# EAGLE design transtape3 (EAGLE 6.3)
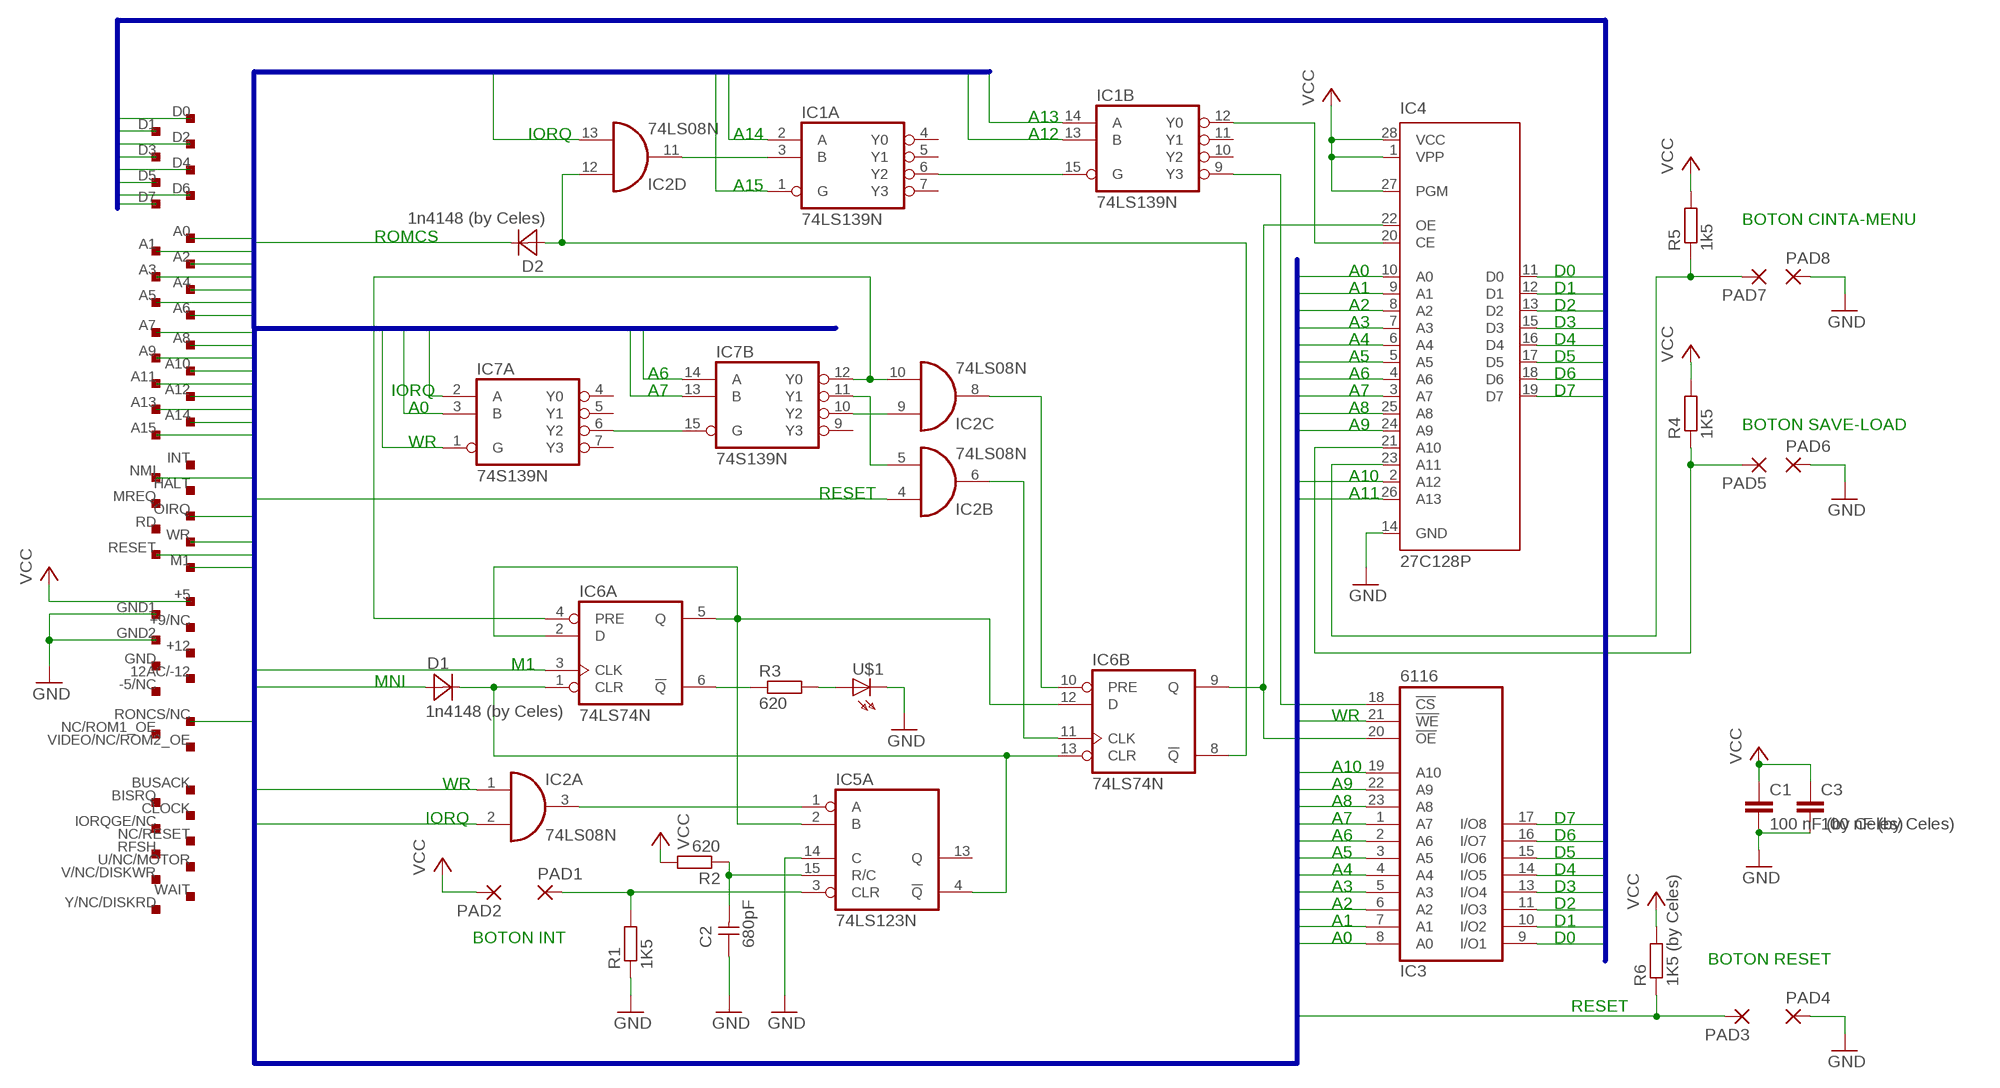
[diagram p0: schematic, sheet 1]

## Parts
C1  100 nF (by Celes)  C-EU050-025X075  [C050-025X075]
C2  680pF  CAPNP-5  [C-5]
C3  100 nF (by Celes)  C-EU050-025X075  [C050-025X075]
D1  1n4148 (by Celes)  DIODE-7,5  [D-7,5]
D2  1n4148 (by Celes)  DIODE-7,5  [D-7,5]
IC1  74LS139N  [DIL16]
IC2  74LS08N  [DIL14]
IC3  6116  6116P  [DIL24-6]
IC4  27C128P  [DIL28-6]
IC5  74LS123N  [DIL16]
IC6  74LS74N  [DIL14]
IC7  74S139N  [DIL16]
PAD1  1,6/0,9  [1,6/0,9]
PAD2  1,6/0,9  [1,6/0,9]
PAD3  1,6/0,9  [1,6/0,9]
PAD4  1,6/0,9  [1,6/0,9]
PAD5  1,6/0,9  [1,6/0,9]
PAD6  1,6/0,9  [1,6/0,9]
PAD7  1,6/0,9  [1,6/0,9]
PAD8  1,6/0,9  [1,6/0,9]
R1  1K5  R-EU_0207/10  [0207/10]
R2  620  R-EU_0207/10  [0207/10]
R3  620  R-EU_0207/10  [0207/10]
R4  1K5  R-EU_0207/10  [0207/10]
R5  1k5  R-EU_0207/10  [0207/10]
R6  1K5 (by Celes)  R-EU_0207/10  [0207/10]
U$1  LED3MM  [LED3MM]
U$2  SPECTRUM_V_1.0  [BUS_SPECTRUM_1.0]

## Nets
A0: IC3.8(A0) IC4.10(A0) IC7.3(A:B) U$2.A0
A1: IC3.7(A1) IC4.9(A1) U$2.A1
A2: IC3.6(A2) IC4.8(A2) U$2.A2
A3: IC3.5(A3) IC4.7(A3) U$2.A3
A4: IC3.4(A4) IC4.6(A4) U$2.A4
A5: IC3.3(A5) IC4.5(A5) U$2.A5
A6: IC3.2(A6) IC4.4(A6) IC7.14(B:A) U$2.A6
A7: IC3.1(A7) IC4.3(A7) IC7.13(B:B) U$2.A7
A8: IC3.23(A8) IC4.25(A8) U$2.A8
A9: IC3.22(A9) IC4.24(A9) U$2.A9
A10: IC3.19(A10) IC4.2(A12) U$2.A10
A11: IC4.26(A13) U$2.A11
A12: IC1.13(B:B) U$2.A12
A13: IC1.14(B:A) U$2.A13
A14: IC1.2(A:A) U$2.A14
A15: IC1.1(A:G) U$2.A15
D0: IC3.9(I/O1) IC4.11(D0) U$2.D0
D1: IC3.10(I/O2) IC4.12(D1) U$2.D1
D2: IC3.11(I/O3) IC4.13(D2) U$2.D2
D3: IC3.13(I/O4) IC4.15(D3) U$2.D3
D4: IC3.14(I/O5) IC4.16(D4) U$2.D4
D5: IC3.15(I/O6) IC4.17(D5) U$2.D5
D6: IC3.16(I/O7) IC4.18(D6) U$2.D6
D7: IC3.17(I/O8) IC4.19(D7) U$2.D7
GND: C1.2 C2.1 C3.2 IC4.14(GND) IC5.14(A:C) PAD4.1(P) PAD6.1(P) PAD8.1(P) R1.1 U$1.K(C) U$2.GND1 U$2.GND2
IORQ: IC2.2(A:I1) IC2.13(D:I1) IC7.2(A:A) U$2.OIRQ
M1: IC6.3(A:CLK) U$2.M1
MNI: D1.1(A) U$2.NMI
N$1: IC1.3(A:B) IC2.11(D:O)
N$2: IC1.6(A:Y2) IC1.15(B:G)
N$3: IC1.9(B:Y3) IC3.18(!CS)
N$4: IC1.12(B:Y0) IC4.20(CE)
N$5: C2.2 IC5.15(A:R/C) R2.1
N$7: IC7.6(A:Y2) IC7.15(B:G)
N$8: IC2.3(A:O) IC5.1(A:A)
N$10: IC5.2(A:B) IC6.2(A:D) IC6.5(A:Q) IC6.12(B:D)
N$11: IC5.3(A:CLR) PAD1.1(P) R1.2
N$12: IC2.5(B:I1) IC7.11(B:Y1)
N$13: IC2.9(C:I0) IC7.10(B:Y2)
N$15: D2.1(A) IC2.12(D:I0) IC6.8(B:!Q)
N$16: IC2.6(B:O) IC6.11(B:CLK)
N$17: D1.2(K) IC5.4(A:!Q) IC6.1(A:CLR) IC6.13(B:CLR)
N$18: IC2.8(C:O) IC6.10(B:PRE)
N$19: IC4.21(A10) PAD5.1(P) R4.1
N$21: IC2.10(C:I1) IC6.4(A:PRE) IC7.12(B:Y0)
N$22: IC6.6(A:!Q) R3.1
N$23: R3.2 U$1.A
N$25: IC3.20(!OE) IC4.22(OE) IC6.9(B:Q)
N$27: IC4.23(A11) PAD7.1(P) R5.1
RESET: IC2.4(B:I0) PAD3.1(P) R6.1 U$2.RESET
ROMCS: D2.2(K) U$2.RONCS/NC
VCC: C1.1 C3.1 IC4.1(VPP) IC4.27(PGM) IC4.28(VCC) PAD2.1(P) R2.2 R4.2 R5.2 R6.2 U$2.+5
WR: IC2.1(A:I0) IC3.21(!WE) IC7.1(A:G) U$2.WR
Unconnected: IC1.4(A:Y0) IC1.5(A:Y1) IC1.7(A:Y3) IC1.10(B:Y2) IC1.11(B:Y1) IC5.5(B:Q) IC5.6(B:C) IC5.7(B:R/C) IC5.9(B:A) IC5.10(B:B) IC5.11(B:CLR) IC5.12(B:!Q) IC5.13(A:Q) IC7.4(A:Y0) IC7.5(A:Y1) IC7.7(A:Y3) IC7.9(B:Y3) U$2.12AC/-12 U$2.+9/NC U$2.+12 U$2.-5/NC U$2.BISRQ U$2.BUSACK U$2.CLOCK U$2.GND U$2.HALT U$2.INT U$2.IORQGE/NC U$2.MREQ U$2.NC/RESET U$2.NC/ROM1_OE U$2.RD U$2.RFSH U$2.U/NC/MOTOR U$2.V/NC/DISKWR U$2.VIDEO/NC/ROM2_OE U$2.WAIT U$2.Y/NC/DISKRD

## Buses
WR,RESET,MNI,M1,IORQ,A[0..15],ROMCS
D[0..7]

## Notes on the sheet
- A13
- IORQ | A14 | A12
- A15
- BOTON CINTA-MENU
- ROMCS
- A0 | D0
- A1 | D1
- A2 | D2
- A3 | D3
- A4 | D4
- A5 | D5
- A6 | A6 | D6
- IORQ | A7 | A7 | D7
- A0 | A8
- A9 | BOTON SAVE-LOAD
- WR
- A10
- RESET | A11
- M1
- MNI
- WR
- A10
- WR | A9
- A8
- IORQ | A7 | D7
- A6 | D6
- A5 | D5
- A4 | D4
- A3 | D3
- A2 | D2
- A1 | D1
- BOTON INT | A0 | D0
- BOTON RESET
- RESET

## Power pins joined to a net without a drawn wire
GND: IC1.8(P:GND) IC2.7(P:GND) IC3.12(GND) IC5.8(P:GND) IC6.7(P:GND) IC7.8(P:GND)
VCC: IC1.16(P:VCC) IC2.14(P:VCC) IC3.24(VCC) IC5.16(P:VCC) IC6.14(P:VCC) IC7.16(P:VCC)

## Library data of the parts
C1 C3 = rcl:C-EU: CAPACITOR, European symbol
C2 = discrete:CAPNP-5
D1 D2 = discrete:DIODE-7,5
IC1 IC7 = 74xx-eu:74*139: Dual 2-line to 4-line DECODER/DEMULTIPLEXER
IC2 = 74xx-eu:74*08: Quad 2-input AND gate
IC3 = memory-idt:6116P: MEMORY
IC4 = microchip:27*128: CMOS EPROM 128 K (16 K x 8)
IC5 = 74xx-eu:74*123: Retriggerable monostable MULTIVIBRATOR
IC6 = 74xx-eu:74*74: Dual D type positive edge triggered FLIP FLOP, preset and clear
PAD1-PAD8 = wirepad:1,6/0,9: THROUGH-HOLE PAD
R1-R6 = rcl:R-EU_: RESISTOR, European symbol
U$1 = led:LED: LED
U$2 = spectrum:SPECTRUM_V_1.0

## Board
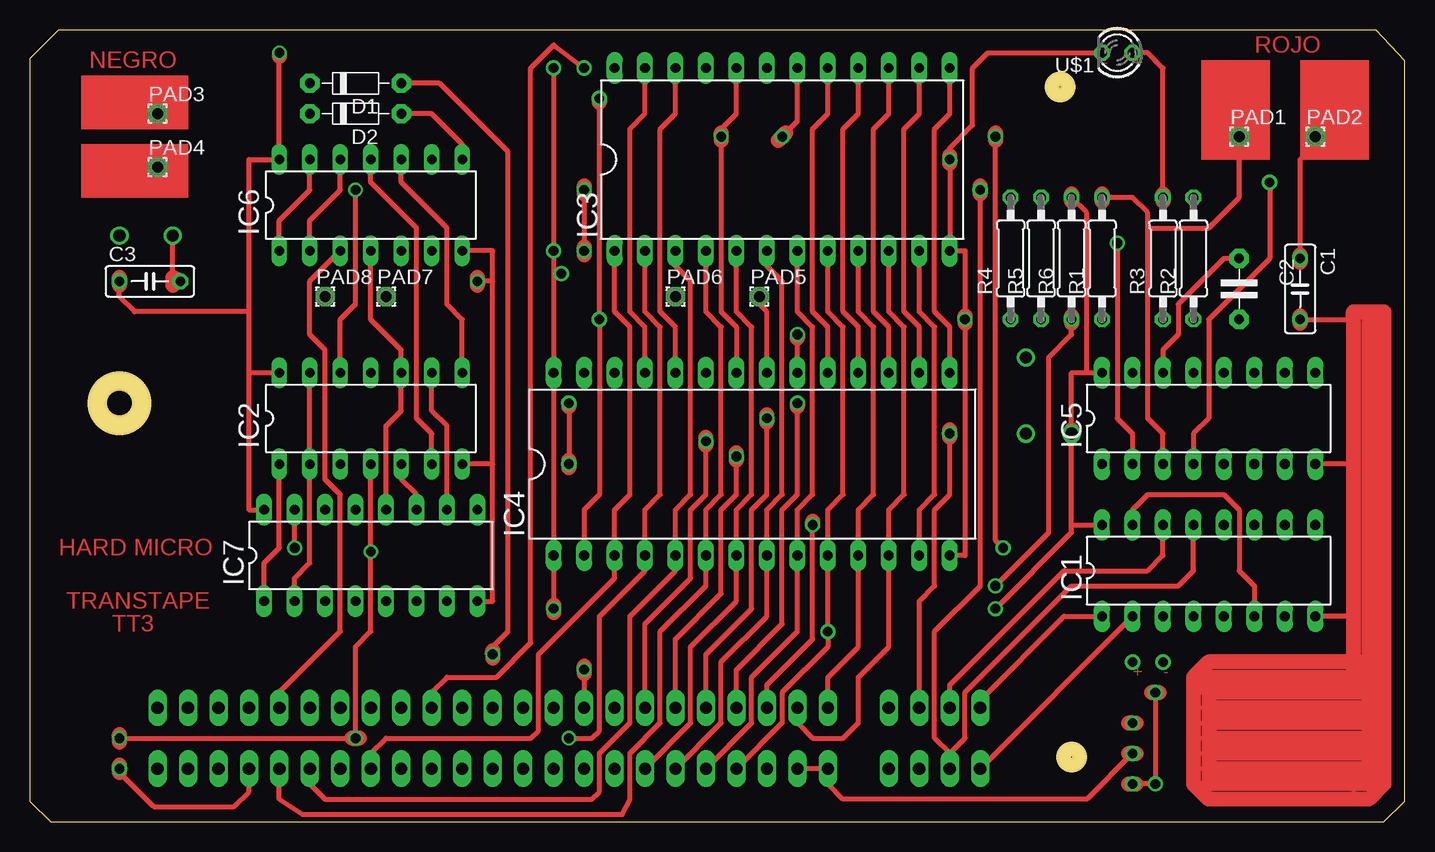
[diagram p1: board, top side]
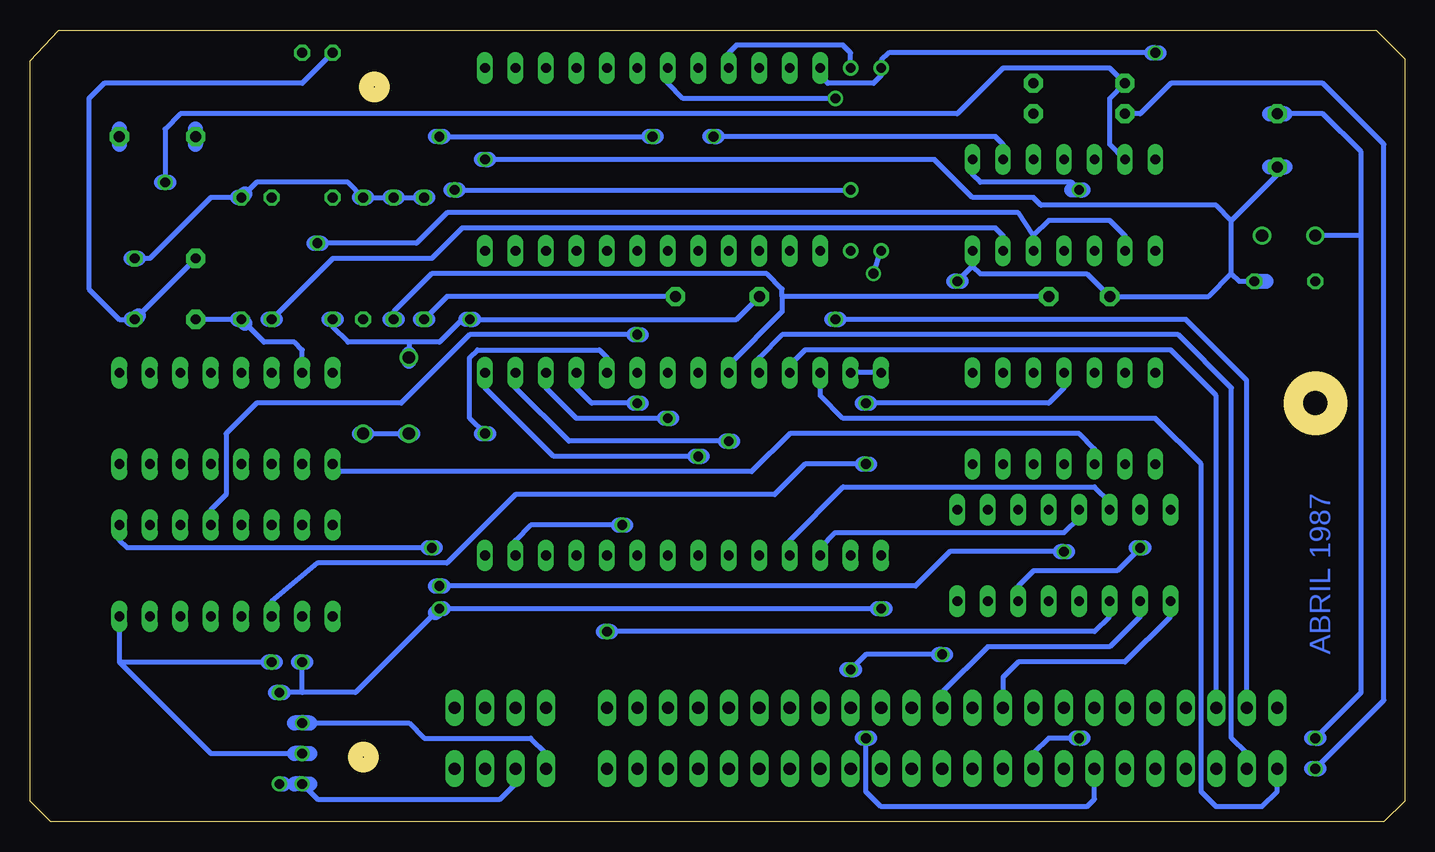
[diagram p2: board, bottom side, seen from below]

Size 114.61 x 66.04 mm. Coordinates in mm from the lower left corner, seen from the top.
Outline: 0,1.74 1.74,0 112.87,0 114.61,1.74 114.61,63.49 112.23,66.04 2.37,66.04 0,63.66 0,1.74
Outline: circle at 86.83,5.4 radius 0.64
Outline: circle at 85.88,61.28 radius 0.64
Outline: circle at 7.46,34.93 radius 1.62
Outline: circle at 7.46,34.93 radius 2.01
Copper layers (1*16): Top 0.035mm / dielectric 1.5mm / Bottom 0.035mm
Design rules "default": minimum track width 10mil, minimum drill 24mil, track to track 8mil, track to pad 8mil, pad to pad 8mil, via to via 8mil, smd to smd 8mil, copper to edge 40mil, drill to drill 8mil, minimum pad ring 10mil, minimum via ring 8mil, stop-mask expansion 4mil, vias tented up to drill 0mil, thermal gap 10mil

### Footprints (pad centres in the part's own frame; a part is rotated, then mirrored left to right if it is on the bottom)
C050-025X075 = drill 0.813 octagon: 1 -2.54,0; 2 2.54,0
C-5 = drill 0.813 pad 1.6 octagon: 1 -2.54,0; 2 2.54,0
D-7,5 = drill 0.813 pad 1.6 octagon: 1 -3.81,0; 2 3.81,0
DIL16 = drill 0.813 long: 1 -8.89,-3.81; 2 -6.35,-3.81; 3 -3.81,-3.81; 4 -1.27,-3.81; 5 1.27,-3.81; 6 3.81,-3.81; 7 6.35,-3.81; 8 8.89,-3.81; 9 8.89,3.81; 10 6.35,3.81; 11 3.81,3.81; 12 1.27,3.81; 13 -1.27,3.81; 14 -3.81,3.81; 15 -6.35,3.81; 16 -8.89,3.81
DIL14 = drill 0.8 long: 1 -7.62,-3.81; 2 -5.08,-3.81; 3 -2.54,-3.81; 4 0,-3.81; 5 2.54,-3.81; 6 5.08,-3.81; 7 7.62,-3.81; 8 7.62,3.81; 9 5.08,3.81; 10 2.54,3.81; 11 0,3.81; 12 -2.54,3.81; 13 -5.08,3.81; 14 -7.62,3.81
DIL24-6 = drill 0.813 long: 1 -13.97,-7.62; 2 -11.43,-7.62; 3 -8.89,-7.62; 4 -6.35,-7.62; 5 -3.81,-7.62; 6 -1.27,-7.62; 7 1.27,-7.62; 8 3.81,-7.62; 9 6.35,-7.62; 10 8.89,-7.62; 11 11.43,-7.62; 12 13.97,-7.62; 13 13.97,7.62; 14 11.43,7.62; 15 8.89,7.62; 16 6.35,7.62; 17 3.81,7.62; 18 1.27,7.62; 19 -1.27,7.62; 20 -3.81,7.62; 21 -6.35,7.62; 22 -8.89,7.62; 23 -11.43,7.62; 24 -13.97,7.62
DIL28-6 = drill 0.813 long: 1 -16.51,-7.62; 2 -13.97,-7.62; 3 -11.43,-7.62; 4 -8.89,-7.62; 5 -6.35,-7.62; 6 -3.81,-7.62; 7 -1.27,-7.62; 8 1.27,-7.62; 9 3.81,-7.62; 10 6.35,-7.62; 11 8.89,-7.62; 12 11.43,-7.62; 13 13.97,-7.62; 14 16.51,-7.62; 15 16.51,7.62; 16 13.97,7.62; 17 11.43,7.62; 18 8.89,7.62; 19 6.35,7.62; 20 3.81,7.62; 21 1.27,7.62; 22 -1.27,7.62; 23 -3.81,7.62; 24 -6.35,7.62; 25 -8.89,7.62; 26 -11.43,7.62; 27 -13.97,7.62; 28 -16.51,7.62
1,6/0,9 = drill 0.914 pad 1.6 octagon: 1 0,0
0207/10 = drill 0.813 octagon: 1 -5.08,0; 2 5.08,0
LED3MM = drill 0.813 octagon: A -1.27,0; K 1.27,0
BUS_SPECTRUM_1.0 = drill 1.016 long: 12AC/-12 12.7,2.54; +5 63.5,-2.54; +9/NC 60.96,-2.54; +12 15.24,2.54; -5/NC 20.32,2.54; A0 48.26,-2.54; A1 45.72,-2.54; A2 43.18,-2.54; A3 40.64,-2.54; A4 10.16,-2.54; A5 12.7,-2.54; A6 15.24,-2.54; A7 17.78,-2.54; A8 5.08,2.54; A9 2.54,-2.54; A10 2.54,2.54; A11 0,-2.54; A12 66.04,-2.54; A13 66.04,2.54; A14 68.58,-2.54; A15 68.58,2.54; BISRQ 22.86,-2.54; BUSACK 5.08,-2.54; CLOCK 50.8,-2.54; D0 55.88,2.54; D1 53.34,2.54; D2 50.8,2.54; D3 43.18,2.54; D4 40.64,2.54; D5 45.72,2.54; D6 48.26,2.54; D7 63.5,2.54; GND 35.56,-2.54; GND1 55.88,-2.54; GND2 53.34,-2.54; HALT 33.02,2.54; INT 38.1,2.54; IORQGE/NC 38.1,-2.54; M1 10.16,2.54; MREQ 30.48,2.54; NC/RESET 0,2.54; NC/ROM1_OE 60.96,2.54; NMI 35.56,2.54; OIRQ 27.94,2.54; RD 25.4,2.54; RESET 20.32,-2.54; RFSH 7.62,2.54; RONCS/NC 7.62,-2.54; U/NC/MOTOR 25.4,-2.54; V/NC/DISKWR 27.94,-2.54; VIDEO/NC/ROM2_OE 33.02,-2.54; WAIT 17.78,2.54; WR 22.86,2.54; Y/NC/DISKRD 30.48,-2.54

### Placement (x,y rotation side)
C1  105.88,44.45 270 top
C2  100.8,44.45 270 top
C3  9.99,45.09 0 top
D1  27.14,61.59 180 top
D2  27.14,59.05 180 top
IC1  98.26,20.95 0 top
IC2  28.41,33.66 0 top
IC3  62.7,55.25 0 top
IC4  60.16,29.84 0 top
IC5  98.26,33.66 0 top
IC6  28.41,51.44 0 top
IC7  28.41,22.22 0 top
PAD1  100.8,57.15 0 top
PAD2  107.15,57.15 0 top
PAD3  10.63,59.05 0 top
PAD4  10.63,54.61 0 top
PAD5  60.8,43.82 0 top
PAD6  53.81,43.82 0 top
PAD7  29.68,43.82 0 top
PAD8  24.6,43.82 0 top
R1  89.37,46.99 90 top
R2  96.99,46.99 90 top
R3  94.45,46.99 90 top
R4  81.75,46.99 90 top
R5  84.29,46.99 90 top
R6  86.83,46.99 90 top
U$1  90.64,64.13 180 top
U$2  10.63,6.99 0 top

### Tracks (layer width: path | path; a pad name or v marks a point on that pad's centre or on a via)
A0  (via drill 0.81 pad 1.27)
  Top 0.406: U$2.A0 62.7,8.26 62.7,10.79 66.51,14.61 v66.51,15.88 IC4.10 66.51,26.04 67.78,27.3 67.78,41.27 66.51,42.55 IC3.8
  Bottom 0.406: 66.19,15.88 25.87,15.88 24.6,17.14 IC7.3
  Bottom 1.27: v66.51,15.88 66.19,15.88 66.83,15.88
A1
  Top 0.406: IC3.7 63.97,42.55 65.24,41.27 65.24,27.3 63.97,26.04 IC4.9 63.97,15.88 60.16,12.06 60.16,8.26 U$2.A1
A2
  Top 0.406: IC3.6 61.43,46.36 62.7,45.09 62.7,27.3 61.43,26.04 IC4.8 61.43,17.14 57.62,13.34 57.62,8.26 U$2.A2
A3
  Top 0.406: IC3.5 58.89,42.55 60.16,41.27 60.16,27.3 58.89,26.04 IC4.7 58.89,18.41 55.08,14.61 55.08,8.26 U$2.A3
A4
  Top 0.406: IC3.4 56.35,42.55 57.62,41.27 57.62,27.3 56.35,26.04 IC4.6 56.35,19.68 52.54,15.88 52.54,8.26 50,5.71 50,1.91 49.37,0.64 22.7,0.64 20.79,1.91 U$2.A4
A5
  Top 0.406: U$2.A5 23.33,3.17 24.6,1.91 46.83,1.91 47.46,2.54 47.46,5.71 50,8.26 50,17.14 53.81,20.95 IC4.5 | IC4.5 53.81,22.86 | IC4.5 53.81,26.04 55.08,27.3 55.08,45.09 53.81,46.36 IC3.3
A6  (via drill 0.81)
  Top 0.406: IC3.2 51.27,42.55 52.54,41.27 52.54,27.3 51.27,26.04 IC4.4 51.27,20.95 47.46,17.14 47.46,7.62 46.83,6.99 v44.92,6.99
  Bottom 0.406: IC7.14 24.6,26.67 25.87,27.94 46.83,27.94 51.27,23.49 IC4.4 | U$2.A6 25.87,1.91 26.5,1.27 43.65,1.27 44.92,2.54 v44.92,6.99
  Bottom 1.27: 44.6,6.99 v44.92,6.99 45.24,6.99
A7
  Top 0.406: IC3.1 48.73,42.55 50,41.27 50,27.3 48.73,26.04 IC4.3 48.73,20.32 42.38,13.97 42.38,7.62 41.75,6.99 29.68,6.99 28.41,5.71 U$2.A7
  Bottom 0.406: IC7.13 27.14,25.4 28.41,24.13 47.46,24.13 48.73,22.86 IC4.3
A8
  Top 0.406: IC3.23 51.27,59.05 50,57.79 50,42.55 51.27,41.27 IC4.25
  Bottom 0.406: IC4.25 51.27,38.1 50,39.37 19.52,39.37 15.71,35.56 U$2.A8
A9
  Top 0.406: IC3.22 53.81,59.05 52.54,57.79 52.54,42.55 53.81,41.27 IC4.24
  Bottom 0.406: IC4.24 53.81,38.73 51.91,40.64 18.88,40.64 14.44,36.2 14.44,6.99 13.17,5.71 U$2.A9
A10  (via drill 0.81 pad 1.27)
  Top 0.406: IC4.2 46.19,26.04 47.46,27.3 v47.46,41.91 47.46,60.01
  Top 1.27: v47.46,60.33 47.46,60.01
  Bottom 0.406: U$2.A10 13.17,36.83 18.25,41.91 47.14,41.91 | IC3.19 61.43,61.59 60.16,60.33 v47.46,60.33
  Bottom 1.27: v47.46,41.91 47.14,41.91 47.78,41.91
A11
  Bottom 0.406: IC4.26 48.73,35.56 46.83,33.66 20.79,33.66 16.98,29.84 16.98,2.54 15.71,1.27 11.9,1.27 10.63,2.54 U$2.A11
A12  (via drill 0.81 pad 1.27)
  Top 0.406: U$2.A12 76.67,5.71 | 76.67,5.71 77.94,6.99 77.94,10.79 86.83,19.68 95.72,19.68 96.99,20.95 IC1.13 | 76.67,5.71 75.4,6.99 75.4,15.88 79.21,19.68 79.21,52.39 v79.21,52.71 | 46.19,52.39 46.19,47.94
  Top 1.27: 46.19,53.02 v46.19,52.71 46.19,52.39 | v46.19,47.62 46.19,47.94 46.19,47.31 | 79.21,53.02 v79.21,52.71 79.21,52.39
  Bottom 0.406: 78.89,52.71 v46.19,52.71
  Bottom 1.27: v79.21,52.71 78.89,52.71 79.53,52.71
A13
  Top 0.406: U$2.A13 76.67,11.43 86.2,20.95 93.18,20.95 94.45,22.22 IC1.14
A14
  Top 0.406: U$2.A14 IC1.2
A15
  Top 0.406: U$2.A15 79.21,10.16 86.2,17.14 IC1.1
D0
  Top 0.406: U$2.D0 66.51,12.06 69.05,14.61 IC4.11 69.05,26.04 70.32,27.3 70.32,41.27 69.05,42.55 IC3.9
D1
  Top 0.406: U$2.D1 63.97,8.26 65.24,6.99 67.78,6.99 69.05,8.26 69.05,12.06 71.59,14.61 IC4.12 71.59,26.04 72.86,27.3 72.86,41.27 71.59,42.55 IC3.10
D2  (via drill 0.81 pad 1.27)
  Top 0.406: U$2.D2 61.43,11.43 65.24,15.24 v65.24,24.76 | IC4.13 74.13,26.04 75.4,27.3 75.4,41.27 74.13,42.55 IC3.11
  Top 1.27: v65.24,24.76 65.24,25.08
  Bottom 0.406: v65.24,24.76 65.56,24.76 72.86,24.76 74.13,23.49 IC4.13
  Bottom 1.27: 64.92,24.76 v65.24,24.76 65.56,24.76
D3  (via drill 0.81 pad 1.27)
  Top 0.406: IC3.13 76.67,59.05 75.4,57.79 75.4,42.55 76.67,41.27 IC4.15 | U$2.D3 53.81,15.24 57.62,19.05 57.62,26.04 58.89,27.3 58.89,30.16 v58.89,30.48
  Top 1.27: 58.89,30.8 v58.89,30.48 58.89,30.16
  Bottom 0.406: IC4.15 76.67,36.2 70.95,30.48 59.21,30.48 v58.89,30.48
  Bottom 1.27: 58.57,30.48 v58.89,30.48 59.21,30.48
D4  (via drill 0.81 pad 1.27)
  Top 0.406: IC3.14 74.13,59.05 72.86,57.79 72.86,42.55 74.13,41.27 IC4.16 | U$2.D4 51.27,16.51 55.08,20.32 55.08,26.04 56.35,27.3 56.35,31.43 v56.35,31.75
  Top 1.27: 56.35,32.07 v56.35,31.75 56.35,31.43
  Bottom 0.406: IC4.16 74.13,36.2 69.69,31.75 56.67,31.75 v56.35,31.75
  Bottom 1.27: 56.03,31.75 v56.35,31.75 56.67,31.75
D5  (via drill 0.81 pad 1.27)
  Top 0.406: IC3.15 71.59,59.05 70.32,57.79 70.32,42.55 71.59,41.27 IC4.17 | U$2.D5 56.35,13.97 60.16,17.78 60.16,26.04 61.43,27.3 61.43,33.34 v61.43,33.66
  Top 1.27: 61.43,33.97 v61.43,33.66 61.43,33.34
  Bottom 0.406: IC4.17 71.59,36.2 69.05,33.66 61.75,33.66 v61.43,33.66
  Bottom 1.27: 61.11,33.66 v61.43,33.66 61.75,33.66
D6  (via drill 0.81 pad 1.27)
  Top 0.406: IC3.16 69.05,59.05 67.78,57.79 67.78,42.55 69.05,41.27 IC4.18 | U$2.D6 58.89,12.7 62.7,16.51 62.7,26.04 63.97,27.3 63.97,34.61
  Top 1.27: v63.97,34.93 63.97,34.61
  Bottom 0.406: IC4.18 69.05,36.2 67.78,34.93 64.29,34.93 v63.97,34.93
  Bottom 1.27: 63.65,34.93 v63.97,34.93 64.29,34.93
D7  (via drill 0.81 pad 1.27)
  Top 0.406: U$2.D7 74.13,18.41 75.4,19.68 75.4,26.04 76.67,27.3 76.67,32.07 v76.67,32.39 | IC3.17 66.51,59.05 65.24,57.79 65.24,42.55 66.51,41.27 IC4.19
  Top 1.27: 76.67,32.7 v76.67,32.39 76.67,32.07
  Bottom 0.406: v76.67,32.39 77.94,33.66 77.94,38.73 77.31,39.37 67.14,39.37 66.51,38.73 IC4.19
  Bottom 1.27: 76.35,32.39 v76.67,32.39 76.99,32.39
GND  (via drill 0.81, 0.81 pad 1.27, 1.02)
  Top 0.406: U$2.GND2 U$2.GND1 66.51,3.17 67.78,1.91 88.1,1.91 v91.91,5.71 | 110.33,17.14 IC1.8 | 110.33,29.84 IC5.8 | C1.2 110.33,41.91 | C2.1 99.53,46.99 95.72,43.18 95.72,40.64 94.45,39.37 IC5.14 | IC4.14 77.94,22.22 77.94,41.59 v77.94,41.91 | 77.94,42.23 77.94,47.62 IC3.12 76.67,54.93 | IC7.8 38.57,18.41 38.57,29.84 | 38.57,29.84 IC2.7 | 38.57,29.84 38.57,45.09 | 38.57,45.09 38.57,47.62 IC6.7 | 38.57,45.09 v37.3,45.09 | U$1.K 79.84,64.13 78.58,62.87 78.58,58.1 76.67,56.2 v76.67,55.25 | 11.9,45.4 v11.9,48.9
  Top 1.27: 98.26,4.45 98.26,3.17 110.33,3.17 | 98.26,6.99 98.26,5.71 | 98.26,9.53 98.26,8.26 | 98.26,10.79 98.26,12.06 110.33,12.06 | 111.59,12.06 110.33,12.06 | 111.59,12.06 111.59,10.79 | 111.59,10.79 111.59,9.53 | 111.59,8.26 111.59,6.99 | 111.59,5.71 111.59,4.45 | 111.59,4.45 111.59,3.17 110.33,3.17 | 111.59,4.45 110.33,3.17 | 111.59,4.45 98.26,4.45 | 98.26,5.71 98.26,4.45 | 111.59,5.71 98.26,5.71 | 111.59,6.99 111.59,5.71 | 111.59,6.99 98.26,6.99 | 98.26,8.26 98.26,6.99 | 111.59,8.26 98.26,8.26 | 111.59,9.53 111.59,8.26 | 111.59,9.53 98.26,9.53 | 98.26,10.79 98.26,9.53 | 111.59,10.79 98.26,10.79 | 110.33,12.06 111.59,10.79 | 110.33,13.34 98.26,13.34 96.99,12.06 96.99,3.17 98.26,1.91 111.59,1.91 112.87,3.17 112.87,13.34 | 110.33,13.34 110.33,17.14 110.33,29.84 110.33,41.91 110.33,42.55 111.59,42.55 | 111.59,42.55 112.87,42.55 112.87,13.34 | 110.33,13.34 110.33,12.06 | 110.33,13.34 112.87,13.34 | 111.59,12.06 112.87,13.34 | 111.59,42.55 111.59,12.06 | 91.59,5.71 v91.91,5.71 92.23,5.71 | v77.94,41.91 77.94,42.23 77.94,41.59 | 76.67,55.56 v76.67,55.25 76.67,54.93 | 37.3,45.4 v37.3,45.09 37.3,44.77 | C3.2 11.9,45.4 11.9,44.77 | 105.88,42.23 C1.2 105.88,41.59
  Bottom 0.406: 92.55,5.71 99.53,5.71 107.15,13.34 | 107.15,13.34 94.45,13.34 | IC1.8 107.15,13.34 | 106.2,41.91 107.15,41.91 109.69,44.45 109.69,60.33 108.42,61.59 91.91,61.59 U$1.K | 105.56,42.23 C2.1 | v37.3,45.09 36.03,46.36 | 36.03,46.36 IC6.7 | 36.03,46.36 35.4,45.72 26.5,45.72 PAD8.1 16.34,43.82 14.44,45.72 | 12.22,45.09 13.8,45.09 14.44,45.72 | 14.44,45.72 14.44,50.16 | 76.35,55.25 39.21,55.25 36.03,52.07 30.95,52.07 30.31,51.44 15.71,51.44 14.44,50.16 | PAD4.1 10.63,53.98 14.44,50.16 | PAD6.1 55.72,41.91 77.62,41.91 | 83.02,40.01 80.48,40.01 78.58,41.91 78.26,41.91 v77.94,41.91 | 83.02,40.01 88.1,40.01 89.37,41.27 R1.1 | 83.02,40.01 83.02,39.05
  Bottom 1.27: 91.28,5.71 v91.91,5.71 92.55,5.71 | 83.02,39.05 v83.02,38.73 83.02,38.42 | v76.67,55.25 76.35,55.25 76.99,55.25 | v77.94,41.91 77.62,41.91 78.26,41.91 | 36.98,45.09 v37.3,45.09 37.62,45.09 | 11.58,45.09 C3.2 12.22,45.09 | 105.56,42.23 C1.2 106.2,41.91 | 89.05,41.91 R1.1 89.69,41.91 | 9.99,54.61 PAD4.1 11.27,54.61
IORQ
  Top 0.406: IC7.2 22.06,20.32 23.33,21.59 IC2.2 IC2.13
  Bottom 0.406: IC7.2 22.06,17.14 24.6,14.61 34.76,14.61 38.57,10.79 U$2.OIRQ
M1
  Top 0.406: U$2.M1 20.79,10.79 25.87,15.88 25.87,27.3 24.6,28.57 24.6,39.37 23.33,40.64 23.33,45.09 IC6.3
MNI  (via drill 0.81)
  Top 0.406: D1.1 34.12,61.59 39.84,55.88 39.84,15.88 38.57,14.61 38.57,14.29 | 46.19,12.38 U$2.NMI
  Top 1.27: 46.19,13.02 v46.19,12.7 46.19,12.38 | v38.57,13.97 38.57,14.29 38.57,13.65
  Bottom 0.406: v38.57,13.97 38.89,13.97 44.92,13.97 v46.19,12.7
  Bottom 1.27: 45.87,12.7 v46.19,12.7 46.51,12.7 | 38.25,13.97 v38.57,13.97 38.89,13.97
N$1  (via drill 0.81 pad 1.27)
  Top 0.406: 44.92,34.61 44.92,30.16
  Top 1.27: v44.92,29.84 44.92,30.16 44.92,29.53 | v44.92,34.93 44.92,34.61
  Bottom 0.406: IC1.3 94.45,18.41 90.64,21.59 79.84,21.59 74.13,27.3 52.54,27.3 50,29.84 45.24,29.84 | 44.6,34.93 29.68,34.93 28.41,36.2 IC2.11
  Bottom 1.27: 44.6,29.84 v44.92,29.84 45.24,29.84 | v44.92,34.93 44.6,34.93 45.24,34.93
N$2
  Top 0.406: IC1.15 91.91,26.04 93.18,27.3 99.53,27.3 100.8,26.04 100.8,20.95 102.07,19.68 IC1.6
N$3  (via drill 0.81 pad 1.27)
  Top 0.406: v81.12,22.86 80.48,23.49 80.48,56.83 | 63.02,57.47 63.97,58.42 IC3.18
  Top 1.27: 80.48,57.47 v80.48,57.15 80.48,56.83 | v62.7,57.15 63.02,57.47 62.38,56.83
  Bottom 0.406: IC1.9 107.15,23.49 106.52,22.86 81.43,22.86 | 80.16,57.15 63.02,57.15 v62.7,57.15
  Bottom 1.27: 80.8,22.86 v81.12,22.86 81.43,22.86 | v80.48,57.15 80.16,57.15 80.8,57.15 | 62.38,57.15 v62.7,57.15 63.02,57.15
N$4  (via drill 0.81 pad 1.27)
  Top 0.406: IC4.20 63.97,40.32
  Top 1.27: v63.97,40.64 63.97,40.32
  Bottom 0.406: IC1.12 99.53,26.04 98.26,27.3 98.26,32.39 95.72,34.93 83.66,34.93 77.94,40.64 64.29,40.64 v63.97,40.64
  Bottom 1.27: 63.65,40.64 v63.97,40.64 64.29,40.64
N$5
  Bottom 0.406: 97.31,41.91 C2.2 | 96.67,41.59 95.09,40.01 92.55,40.01 91.91,39.37 IC5.15
  Bottom 1.27: 97.31,41.91 R2.1 96.67,41.59
N$6  (via drill 0.81)
  Top 1.27: 91.59,8.26 v91.91,8.26 92.23,8.26
  Bottom 0.406: 91.28,8.26 83.02,8.26 81.75,6.99 72.86,6.99 71.59,5.71
  Bottom 1.27: v91.91,8.26 91.28,8.26 92.55,8.26
N$7  (via drill 0.81 pad 1.27)
  Top 0.406: v22.06,22.86 IC7.15
  Bottom 0.406: IC7.6 32.22,19.68 30.95,20.95 23.96,20.95 v22.06,22.86
  Bottom 1.27: 21.74,22.86 v22.06,22.86 22.38,22.86
N$8
  Bottom 0.406: IC5.1 88.73,29.21 54.45,29.21 51.27,32.39 27.14,32.39 25.87,31.11 IC2.3
N$10  (via drill 0.81 pad 1.27)
  Top 0.406: IC5.2 91.91,32.39 90.64,33.66 v90.64,48.26 | IC6.2 23.33,50.16 25.87,52.71 IC6.12
  Bottom 0.406: 90.32,48.26 82.39,48.26 79.84,50.8 32.22,50.8 30.95,48.9 | 30.95,48.9 IC6.5 | 30.95,48.9 29.68,50.16 24.6,50.16 23.33,48.9 IC6.2
  Bottom 1.27: v90.64,48.26 90.32,48.26 90.96,48.26
N$11
  Top 0.406: PAD1.1 100.8,52.07 98.26,49.53 93.18,49.53 | R1.2 91.91,52.07 93.18,50.8 93.18,49.53 | 93.18,49.53 93.18,33.66 94.45,32.39 IC5.3
  Top 1.27: 89.37,52.39 R1.2 89.37,51.75
  Bottom 1.27: 100.8,57.79 PAD1.1 100.8,56.52
N$12
  Top 0.406: IC2.5 30.95,28.57 32.22,27.3 IC7.11
N$13
  Top 0.406: IC7.10 34.76,33.02 33.49,34.29 IC2.9
N$15  (via drill 0.81)
  Top 0.406: D2.1 33.49,59.05 36.03,56.52 IC6.8 | v27.14,52.71 27.14,43.18 25.87,41.91 IC2.12
  Bottom 0.406: IC6.8 36.03,53.98 35.4,53.34 27.77,53.34 v27.14,52.71
  Bottom 1.27: 26.82,52.71 v27.14,52.71 27.77,52.71
N$16
  Top 0.406: IC2.6 33.49,32.39 32.22,33.66 32.22,49.53 28.41,53.34 IC6.11
N$17  (via drill 0.81 pad 1.27)
  Top 0.406: IC5.4 96.99,32.39 98.26,33.66 98.26,41.91 103.34,46.99 v103.34,53.34 | IC6.13 23.33,52.71 20.79,50.16 IC6.1
  Bottom 0.406: v103.34,53.34 103.34,57.79 102.07,59.05 37.3,59.05 33.49,62.87 24.6,62.87 D1.2 24.6,60.33 24.6,56.52 IC6.13
  Bottom 1.27: 103.02,53.34 v103.34,53.34 103.66,53.34
N$18
  Top 0.406: IC2.8 36.03,41.91 34.76,43.18 34.76,49.53 30.95,53.34 IC6.10
N$19
  Top 0.406: IC4.21 61.43,42.55 60.8,43.18 PAD5.1
  Bottom 0.406: R4.1 79.84,43.82 PAD5.1
  Bottom 1.27: 81.43,41.91 R4.1 82.07,41.91
N$21
  Top 0.406: IC6.4 28.41,41.91 30.95,39.37 IC2.10 30.95,34.29 29.68,33.02 IC7.12
N$22
  Bottom 0.406: IC6.6 33.49,48.9 34.12,49.53 78.58,49.53 81.12,46.99 89.37,46.99 R3.1
  Bottom 1.27: 94.13,41.91 R3.1 94.77,41.91
N$23
  Top 0.406: 94.45,52.39 94.45,62.87 93.18,64.13 U$1.A
  Top 1.27: 94.45,52.39 R3.2 94.45,51.75
N$25  (via drill 0.81)
  Top 0.406: IC3.20 58.89,59.05 57.62,57.79 57.62,57.47 | v57.62,57.15 57.62,56.83 57.62,42.55 58.89,41.27 IC4.22
  Top 1.27: v57.62,57.15 57.62,57.47 57.62,56.83
  Bottom 0.406: IC6.9 33.49,56.52 34.12,57.15 57.3,57.15
  Bottom 1.27: v57.62,57.15 57.3,57.15 57.94,57.15
N$27
  Bottom 0.406: PAD7.1 51.91,43.82 | 51.91,43.82 51.91,42.55 56.35,38.1 IC4.23 | R5.1 84.29,42.55 81.12,45.72 53.18,45.72 51.91,44.45 51.91,43.82
  Bottom 1.27: 83.97,41.91 R5.1 84.61,41.91
N$28  (via drill 0.81 pad 1.27)
  Bottom 1.27: 91.59,13.34 v91.91,13.34 92.23,13.34
N$29  (via drill 0.81 pad 1.27)
  Bottom 1.27: 94.13,13.34 v94.45,13.34 94.77,13.34
RESET  (via drill 0.81, 1.02)
  Top 0.406: v27.14,6.99 27.14,14.61 28.41,15.88 v28.41,22.54 IC2.4 | v7.46,6.99 26.82,6.99 | 86.83,41.59 86.83,40.64 84.92,38.73 84.92,24.13 v80.48,19.68
  Top 1.27: v27.14,6.99 26.82,6.99 27.46,6.99 | 7.46,7.3 v7.46,6.99 7.46,6.67 | 86.83,42.23 R6.1 86.83,41.59
  Bottom 0.406: U$2.RESET 30.95,5.71 29.68,6.99 27.46,6.99 | 9.99,59.05 6.82,59.05 3.64,55.88 3.64,48.9 | 3.64,48.9 3.64,10.79 v7.46,6.99 | 3.64,48.9 v7.46,48.9 | 80.16,19.68 40.79,19.68 37.94,22.54 28.73,22.54
  Bottom 1.27: 7.77,6.99 v7.46,6.99 7.14,6.99 | 26.82,6.99 v27.14,6.99 27.46,6.99 | v80.48,19.68 80.16,19.68 80.8,19.68 | 28.09,22.54 v28.41,22.54 28.73,22.54 | PAD3.1 9.99,59.05 11.27,59.05
ROMCS  (via drill 0.81 pad 1.27)
  Top 0.406: U$2.RONCS/NC 18.25,2.54 16.98,1.27 10.31,1.27 7.46,4.13
  Top 1.27: 7.46,4.76 v7.46,4.45 7.46,4.13
  Bottom 0.406: v7.46,4.45 1.74,10.16 1.74,56.52 6.82,61.59 19.52,61.59 22.06,59.05 D2.2
  Bottom 1.27: 7.77,4.45 v7.46,4.45 7.14,4.45
VCC  (via drill 0.81, 0.81 pad 1.27, 1.02)
  Top 0.406: 92.23,3.17 v93.81,3.17 v93.81,10.79 | v80.48,17.78 86.83,24.13 86.83,24.76 | 86.83,24.76 IC1.16 | 86.83,24.76 86.83,32.07 v86.83,32.39 | 86.83,32.7 86.83,37.47 88.1,37.47 | 88.1,37.47 IC5.16 | 105.88,47.31 105.88,55.25 107.15,56.52 PAD2.1 | 88.1,37.47 88.1,50.8 R6.2 | 43.65,18.1 IC4.1 IC4.28 43.65,45.72 | 43.65,45.72 v43.65,47.62 v43.65,62.87 | 43.65,45.72 v44.29,45.72 | IC7.16 18.25,26.04 18.25,37.47 | 18.25,37.47 IC2.14 | 18.25,37.47 18.25,42.55 | 18.25,42.55 8.72,42.55 7.46,43.82 7.46,44.77 | 18.25,42.55 18.25,55.25 IC6.14 20.79,63.82
  Top 1.27: v43.65,17.78 43.65,18.1 43.65,17.46 | 91.59,3.17 v91.91,3.17 92.23,3.17 | 93.5,10.79 v93.81,10.79 94.13,10.79 | v86.83,32.39 86.83,32.7 86.83,32.07 | v20.79,64.13 20.79,63.82 | 7.46,45.4 C3.1 7.46,44.77 | C1.1 105.88,47.31 105.88,46.67 | 86.83,52.39 R6.2 86.83,51.75
  Bottom 0.406: U$2.+5 74.13,3.17 75.4,1.91 90.64,1.91 v91.91,3.17 | 91.91,10.79 93.5,10.79 | 91.91,10.79 91.91,13.34 | 91.91,10.79 87.47,10.79 80.8,17.46 | 97.31,52.07 99.53,52.07 104.61,46.99 105.56,46.99 | 96.67,52.39 95.72,53.34 88.1,53.34 R6.2 | 43.97,17.78 80.16,17.78 | IC4.28 IC4.27 | IC3.24 48.73,62.23 48.09,61.59 44.29,61.59 43.65,62.23 v43.65,62.87 43.65,63.5 43.02,64.13 21.11,64.13 | 83.97,52.07 82.07,52.07 | 86.51,52.07 84.61,52.07 R5.2 | 86.51,32.39 83.34,32.39 | 92.55,3.17 93.5,3.17 | v44.29,45.72 v43.65,47.62
  Bottom 1.27: 43.33,17.78 v43.65,17.78 43.97,17.78 | 91.28,3.17 v91.91,3.17 92.55,3.17 | v93.81,3.17 93.5,3.17 | 93.5,10.79 v93.81,10.79 94.13,10.79 | 80.16,17.78 v80.48,17.78 80.8,17.46 | 82.7,32.39 v83.02,32.39 83.34,32.39 | v86.83,32.39 86.51,32.39 87.15,32.39 | 20.47,64.13 v20.79,64.13 21.11,64.13 | C1.1 105.56,46.99 106.2,46.99 | 96.67,52.39 R2.2 97.31,52.07 | 81.43,52.07 R4.2 82.07,52.07 | R5.2 83.97,52.07 84.61,52.07 | R6.2 86.51,52.07 87.15,52.07 | 107.15,57.79 PAD2.1 107.15,56.52
WR  (via drill 0.81 pad 1.27)
  Top 0.406: IC7.1 19.52,21.59 20.79,22.86 IC2.1 | v46.19,62.87 43.65,64.77 41.75,62.87 41.75,14.92 38.89,12.06 34.76,12.06 33.49,10.79 U$2.WR
  Bottom 0.406: IC7.1 19.52,17.14 23.33,13.34 32.22,13.34 33.49,12.06 U$2.WR | v46.19,62.87 46.19,64.13 46.83,64.77 55.72,64.77 56.35,64.13 IC3.21
(copper drawn outside any net)
  shapes: Top area x8

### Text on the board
Top: ROJO | NEGRO | - | + | HARD MICRO | TRANSTAPE | TT3 | + | -
Bottom: ABRIL 1987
